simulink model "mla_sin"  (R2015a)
settings: Solver=FixedStepDiscrete  StartTime=0.0  StopTime=10  FixedStep=0.0001  RelTol=1e-3
PreLoadFcn:
  | MLA_Sensor1 = load('mla_sensor1.dat');
libraries: libmla x1, slrtlib x1

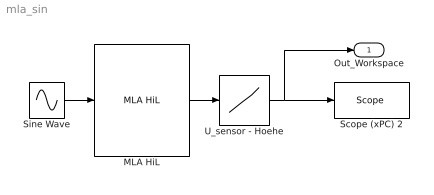
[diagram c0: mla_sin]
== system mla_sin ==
  MLA HiL : libmla/MLA HiL  SystemSampleTime=-1
  Scope (xPC) 2 : slrtlib/Displays and Logging/Scope   scopeno=1  scopetype=Target  autostart=on  viewmode=Graphical sliding  formatstr='%15.6f'  grid=on  ylimits=[0 0.132]  nosamples=1000  noprepostsamples=0  interleave=10  triggermode=FreeRun  triggersignal=1  trigsignalfromport=off  triggerlevel=0.0  triggerslope=Either  triggerscope=1  triggersample=0  filename=data.dat  mode=Lazy  writesize=512  autorestart=off  dynamicfilemode=off  maxwritefilesize=512*1024^2
  Sine Wave : Sin  Bias=2.5  Frequency=2  SampleTime=0
  U_sensor - Hoehe : Lookup  InputValues=MLA_Sensor1(:,1)  Table=MLA_Sensor1(:,2)
  Out_Workspace : Outport
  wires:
  U_sensor - Hoehe/1 -> Out_Workspace/1, Scope (xPC) 2/1
  Sine Wave/1 -> MLA HiL/1
  MLA HiL/1 -> U_sensor - Hoehe/1
